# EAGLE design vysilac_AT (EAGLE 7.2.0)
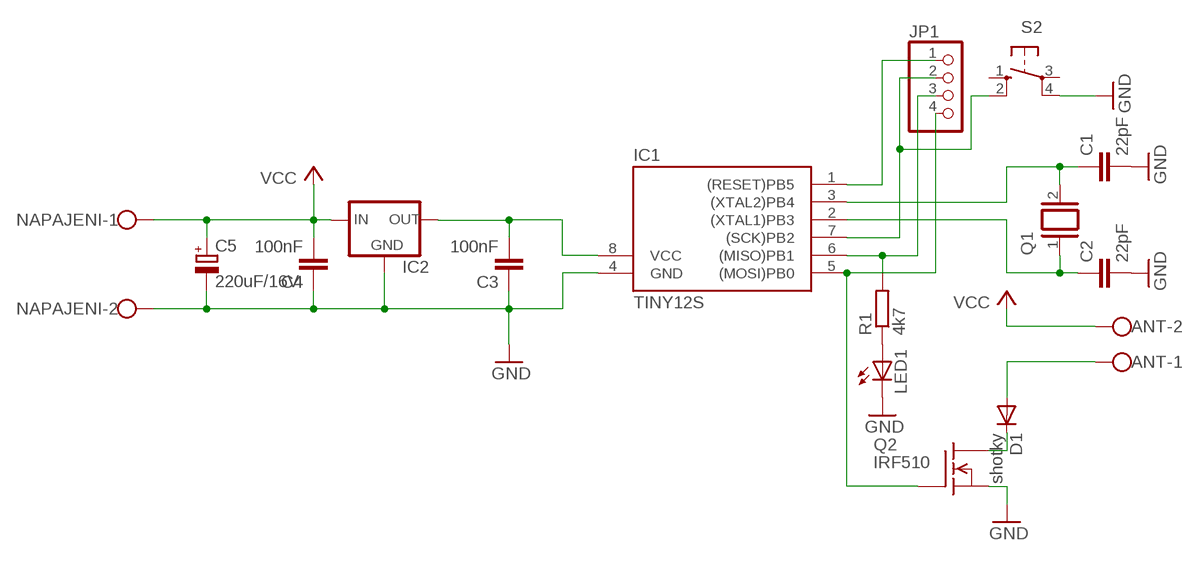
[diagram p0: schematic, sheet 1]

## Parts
ANT  W237-102  [W237-102]
C1  22pF  C-EUC0805K  [C0805K]
C2  22pF  C-EUC0805K  [C0805K]
C3  100nF  C-EUC0805K  [C0805K]
C4  100nF  C-EUC0805K  [C0805K]
C5  220uF/16V  CPOL-EUE2.5-5  [E2,5-5]
D1  shotky  DIODE-DO27-15  [DO27-15]
IC1  TINY12S  [SOIC8]
IC2  78LXX  [78LXX]
JP1  PINHD-1X4  [1X04]
LED1  LED3MM  [LED3MM]
NAPAJENI  W237-102  [W237-102]
Q1  XTAL/S  [QS]
Q2  IRF510  [TO220]
R1  4k7  R-EU_R0805  [R0805]
S2  10-XX  [B3F-10XX]

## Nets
GND: C1.2 C2.2 C3.1 C4.1 C5.- IC1.4(GND) IC2.GND LED1.K(C) NAPAJENI.2 Q2.3(S) S2.4(P1)
N$1: C1.1 IC1.3((XTAL2)PB4) Q1.2
N$2: C2.1 IC1.2((XTAL1)PB3) Q1.1
N$3: IC1.5((MOSI)PB0) JP1.4 Q2.1(G)
N$4: C3.2 IC1.8(VCC) IC2.OUT
N$6: LED1.A R1.1
N$7: D1.C Q2.2(D)
N$8: ANT.1 D1.A
N$9: IC1.1((RESET)PB5) JP1.1
N$10: IC1.7((SCK)PB2) JP1.2 S2.2(S1)
N$11: IC1.6((MISO)PB1) JP1.3 R1.2
VCC: ANT.2 C4.2 C5.+ IC2.IN NAPAJENI.1
Unconnected: S2.1(S) S2.3(P)

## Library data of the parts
ANT NAPAJENI = con-wago-500:W237-102: WAGO SCREW CLAMP
C1-C4 = rcl:C-EU: CAPACITOR, European symbol
C5 = rcl:CPOL-EU: POLARIZED CAPACITOR, European symbol
D1 = diode:DIODE-: DIODE
IC1 = atmel:TINY12*: MICROCONTROLLER 1 Kbytes FLASH 64 bytes EEPROM
IC2 = v-reg:78LXX: VOLTAGE REGULATOR
JP1 = pinhead:PINHD-1X4: PIN HEADER
LED1 = led:LED: LED
Q1 = special:XTAL/S: CRYSTAL
Q2 = transistor-fet:IRF510: N-Channel Enhancement MOSFET (HEXFET); 100V; 5,6A; 0,54Ohm
R1 = rcl:R-EU_: RESISTOR, European symbol
S2 = switch-omron:10-XX: OMRON SWITCH; MPN: B3F-1000; OC_FARNELL: 176432; OC_NEWARK: 36M3542

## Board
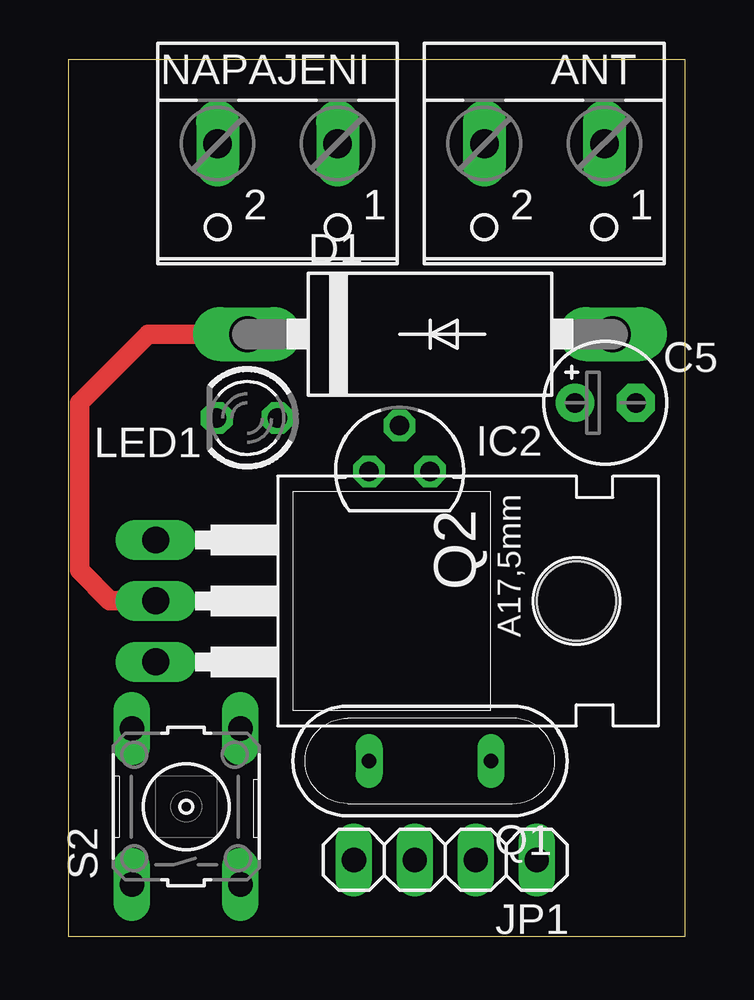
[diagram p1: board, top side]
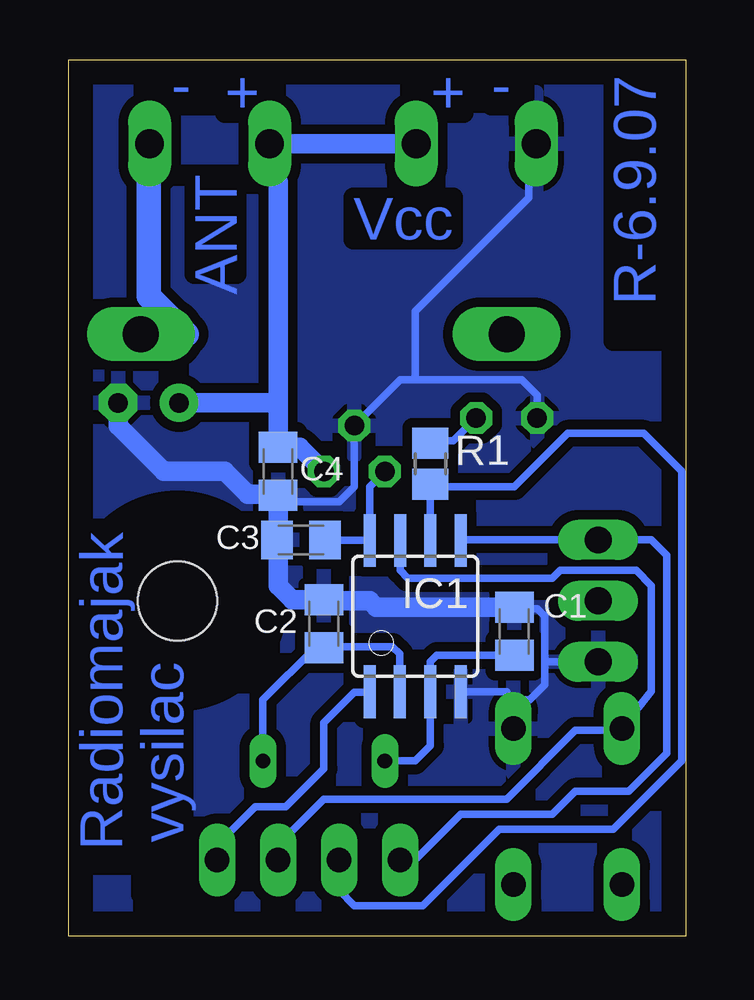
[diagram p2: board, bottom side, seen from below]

Size 25.7 x 36.5 mm. Coordinates in mm from the lower left corner, seen from the top.
Outline: 0,0 25.7,0 25.7,36.5 0,36.5 0,0
Copper layers (1*16): Top 0.035mm / dielectric 1.5mm / Bottom 0.035mm
Design rules "default": minimum track width 10mil, minimum drill 24mil, track to track 8mil, track to pad 8mil, pad to pad 8mil, via to via 8mil, smd to smd 8mil, copper to edge 40mil, drill to drill 8mil, minimum pad ring 10mil, minimum via ring 8mil, stop-mask expansion 4mil, vias tented up to drill 0mil, thermal gap 10mil

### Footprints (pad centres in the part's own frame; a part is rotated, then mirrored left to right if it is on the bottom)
W237-102 = drill 1.194 long: 1 -2.5,-1.27; 2 2.5,-1.27
C0805K = smd 1.3 x 1.6: 1 -1,0; 2 1,0
E2,5-5 = drill 0.813 pad 1.6: + -1.27,0 | drill 0.813 pad 1.6 octagon: - 1.27,0
DO27-15 = drill 1.499 long: A 7.62,0; C -7.62,0
SOIC8 = smd 0.5 x 2.2: 1 -1.905,-3.154; 2 -0.645,-3.154; 3 0.625,-3.154; 4 1.895,-3.154; 5 1.905,3.154; 6 0.635,3.154; 7 -0.635,3.154; 8 -1.905,3.154
78LXX = drill 0.813 octagon: GND 0,1.905; IN 1.27,0; OUT -1.27,0
1X04 = drill 1.016 long: 1 -3.81,0; 2 -1.27,0; 3 1.27,0; 4 3.81,0
LED3MM = drill 0.813 octagon: A -1.27,0; K 1.27,0
QS = drill 0.61 long: 1 -2.54,0; 2 2.54,0
TO220 = drill 1.118 long: 1 -2.54,-6.35; 2 0,-6.35; 3 2.54,-6.35 | hole 3.302: 0,11.176
R0805 = smd 1.3 x 1.5: 1 -0.85,0; 2 0.85,0
B3F-10XX = drill 1.016 long: 1 -3.251,2.261; 2 3.251,2.261; 3 -3.251,-2.261; 4 3.251,-2.261

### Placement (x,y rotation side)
ANT  19.84,31.75 180 top
C1  7.14,12.7 90 bottom
C2  15.07,13.01 90 bottom
C3  16.03,16.5 0 bottom
C4  16.98,19.36 90 bottom
C5  22.38,22.22 0 top
D1  15.07,25.08 0 top
IC1  11.27,13.33 0 bottom
IC2  13.8,19.36 0 top
JP1  15.71,3.17 180 top
LED1  7.46,21.59 180 top
NAPAJENI  8.72,31.75 180 top
Q1  15.07,7.3 180 top
Q2  9.99,13.96 270 top
R1  10.63,19.68 270 bottom
S2  4.92,5.39 90 top

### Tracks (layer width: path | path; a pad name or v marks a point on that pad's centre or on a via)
GND
  Bottom 0.305: 5.87,11.43 5.87,10.47 6.5,9.84 7.16,9.84 7.18,9.82 | 5.87,11.43 5.87,13.33 6.18,13.65 7.14,13.65 C1.2 | 7.14,13.96 7.18,14.01 7.77,14.01 7.77,13.96 | 16.98,18.41 17.03,18.36 | C4.1 16.61,18.36 16.34,18.09 14.44,18.09 13.8,18.73 IC2.GND 11.9,23.17 11.27,23.17 | Q2.3 5.87,11.43 | 7.49,10.14 7.46,10.18 | LED1.K 6.18,22.54 6.82,23.17 11.27,23.17 | 6.54,32.98 6.54,30.75 11.27,26.03 11.27,23.17 | IC1.4 7.53,10.18 7.49,10.14 | S2.4 7.18,9.82 | 7.18,9.82 7.49,10.14
  Bottom 0.61: 6.54,32.98 6.22,32.98
  Bottom 0.813: C5.- 23.65,21.27 21.74,19.36 19.2,19.36 18.25,18.41 16.98,18.41 C4.1 16.98,16.5 | C1.2 12.9,13.7 13.17,13.96 15.07,13.96 C2.2 16.39,14.01 16.98,14.6 16.98,16.5 | 16.98,16.5 C3.1
  pour Bottom (isolate 0.406): -0.17,36.83 -0.17,4.76 0.15,-0.64 26.19,-0.64 26.5,4.12 26.5,35.87 25.55,36.83
N$1
  Bottom 0.305: 10.63,10.16 10.63,7.93 11.27,7.3 Q1.2 | C1.1 10.36,11.7 10.63,11.43 10.63,10.16 | 10.63,10.16 IC1.3
N$2
  Bottom 0.305: IC1.2 11.91,11.75 12.22,12.06 15.03,12.06 C2.1 15.44,12.01 17.61,9.84 Q1.1
N$3
  Bottom 0.305: IC1.5 9.36,16.5 Q2.1 1.42,16.5 0.79,15.87 0.79,7.62 2.38,6.03 4.6,6.03 5.55,5.08 9.36,5.08 11.27,3.17 JP1.4
N$4
  Bottom 0.305: IC2.OUT 13.17,18.73 IC1.8 15.05,16.48 15.07,16.5 C3.2
N$6
  Bottom 0.305: R1.1 10.53,20.53 10.31,20.32 10.31,20.63 9.68,20.63 LED1.A
N$7
  Top 0.813: Q2.2 1.74,13.96 0.47,15.23 0.47,22.22 3.33,25.08 D1.C
N$8
  Bottom 1.016: D1.A 20.79,25.08 22.38,26.66 22.38,33.02 ANT.1
N$9
  Bottom 0.305: JP1.1 19.52,3.81 17.93,5.39 16.66,5.39 15.07,6.98 15.07,8.88 13.8,10.16 13.19,10.16 IC1.1
N$10
  Bottom 0.305: JP1.2 16.98,3.81 15.07,5.71 7.46,5.71 4.6,8.57 3.05,8.57 S2.2 1.42,10.19 1.42,14.6 2.06,15.23 5.23,15.23 5.55,14.92 11.58,14.92 11.9,15.23 IC1.7
N$11
  Bottom 0.305: IC1.6 R1.2 10.53,18.73 7.14,18.73 4.92,20.95 1.74,20.95 0.15,19.36 0.15,7.3 3.01,4.44 7.77,4.44 10.95,1.27 13.8,1.27 14.44,1.9 JP1.3
VCC
  Bottom 0.305: C4.2 16.07,20.36
  Bottom 0.813: NAPAJENI.1 ANT.2 17.34,31.79 16.98,31.43 16.98,22.22 | 16.98,20.32 C4.2 16.98,22.22 | 16.98,22.22 C5.+ | 16.07,20.36 IC2.IN

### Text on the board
Bottom: R-6.9.07 | - | - | + | + | ANT | Vcc | Radiomajak | vysilac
